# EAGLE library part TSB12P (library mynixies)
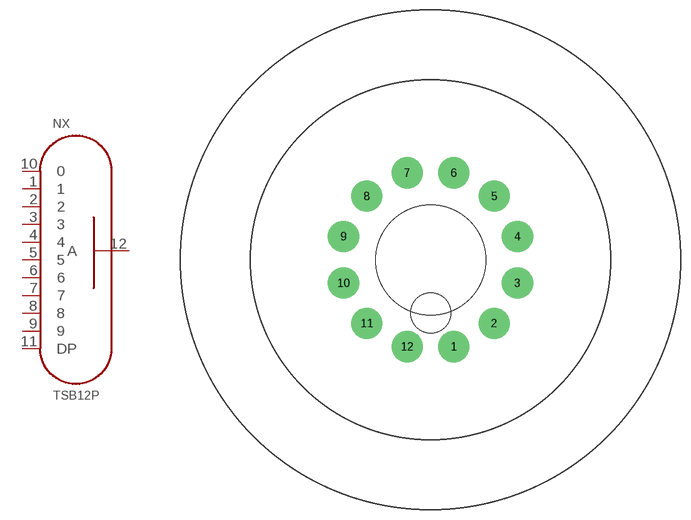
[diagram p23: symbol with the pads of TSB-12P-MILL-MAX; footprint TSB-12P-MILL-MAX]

Designator prefix NX

## TSB12P  [TSB-12P-MILL-MAX]
1  1  pas
2  2  pas
3  3  pas
4  4  pas
5  5  pas
6  6  pas
7  7  pas
8  8  pas
9  9  pas
10  0  pas
11  DP  pas
12  A  pas

## Footprint TSB-12P-MILL-MAX (pad centres in mm)
drill 3.66: 1 3.494,-13.04; 2 9.546,-9.546; 3 13.04,-3.494; 4 13.04,3.494; 5 9.546,9.546; 6 3.494,13.04; 7 -3.494,13.04; 8 -9.546,9.546; 9 -13.04,3.494; 10 -13.04,-3.494; 11 -9.546,-9.546; 12 -3.494,-13.04
hole 16.5 at 0,0
hole 6 at 0,-8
